PROGRAM Main_CM
VAR CONSTANT
	cInitEnvSpec 	: ST_CM_EnvelopeSpectrum_InitPars := (	nFFT_Length			:= cFFTLength,
															nWindowLength		:= cWindowLength,
															bTransformToDecibel	:= FALSE,
															fDecibelThreshold	:= cCM_MinArgLog10, 
															eWindowType			:= eCM_HannWindow,           
															eScalingType 		:= eCM_RMS);               															
END_VAR
VAR	
	fbEnvSpec			: FB_CMA_EnvelopeSpectrum :=( stInitPars := cInitEnvSpec, nOwnID := eID_EnvSpec, aDestIDs := [eID_Sink] );														
	fbErrHist			: FB_HRErrHist; // error monitoring
END_VAR


// Call Envelope Spectrum 
fbEnvSpec.Call();
IF fbEnvSpec.bError THEN
	fbErrHist.AddError(bErr:=TRUE, hrErrCode:=fbEnvSpec.hrErrorCode, sErrSource:='MAIN_CM.fbEnvSpec'); // error monitoring
	// ToDo: if error
END_IF

END_PROGRAM
